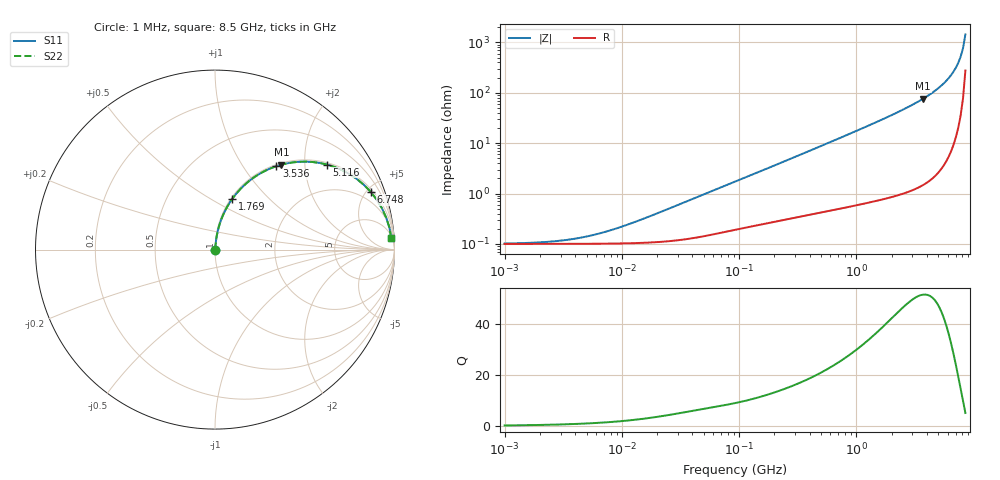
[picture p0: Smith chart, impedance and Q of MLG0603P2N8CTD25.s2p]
! S-Parameter Data Generated by TDK Corporation
! Copyright(C) 2025 TDK Corporation.
! All Rights Reserved.
! TDK P/N: MLG0603P2N8CTD25 (SMD / SMT Inductor (Coil))
! Property: L=2.8nH at 500MHz
! Size(LxWxT): 0.6x0.3x0.3mm
! Model Type: s2p (Touchstone File Format Version 1.0)
! Frequency: DC=Yes Start=1MHz Stop=8500MHz 198points Log-sweep
! Model Generated on Feb. 6, 2025
! Terms and conditions regarding TDK Simulation Models:
! 1)This simulation model is being provided solely for informational
!  purposes. Please refer to the specifications of the products in
!  terms of detailed characteristics of such products.
! 2)In no event shall TDK Corporation of any of its subsidiaries be
!  liable for any loss or damage arising, directly or indirectly,
!  from any information contained in this simulation model, including,
!  but not limited to loss or damages arising from any inaccuracies,
!  omissions or errors in connection with such information.
! 3)Any and all copyrights on this simulation model are owned by
!  TDK Corporation.  Duplication or redistribution of this simulation
!  model without prior written permission from TDK Corporation
!  is prohibited.
! 4)This simulation model is subject to any modification or change
!  without any prior notice.
! 5)Neither TDK Corporation nor any of its subsidiaries shall make any
!  warranty, express or implied, including but not limited to the
!  correctness, implied warranties of merchantability and fitness for
!  a particular purpose with respect to this simulation models.
! 6)The use of this simulation model shall be deemed to have consented
!  to the terms and conditions hereof.
! Port Assignments:
!  1 ---@@@--- 2
! Applicable Conditions:
!  Temperature = 25 degC
!  DC Bias Current = 0 A
!  Small Signal Operation
# Hz S MA R 50
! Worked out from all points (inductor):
!   197 points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, 1 MHz to 8.5 GHz, reference 50 ohm
!   read as one part in series: L = 3.1 nH near 16.71 MHz
!   highest Q = 51.7 at 3.703 GHz (marker M1), where L = 3.28 nH
!   S11 on the Smith chart (normalised r, x): 1 MHz: 1.00, +0.00; 1.769 GHz: 1.02, +0.63; 3.536 GHz: 1.03, +1.43; 5.116 GHz: 1.06, +2.59; 6.748 GHz: 1.19, +5.31; 8.5 GHz: 7, +28
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1000000  0.001018 11.1  0.999 -0.0  0.999 -0.0  0.001018 11.1
2403882  0.001105 25.1  0.999 -0.0  0.999 -0.0  0.001105 25.1
4587603  0.001346 41.7  0.999 -0.1  0.999 -0.1  0.001346 41.7
6337562  0.001597 50.8  0.999 -0.1  0.999 -0.1  0.001597 50.8
8755050  0.00199 59.2  0.999 -0.1  0.999 -0.1  0.00199 59.2
2.10461e7  0.004237 74.8  0.9989 -0.2  0.9989 -0.2  0.004237 74.8
9.219544e7  0.01721 82.7  0.998 -1.0  0.998 -1.0  0.01721 82.7
4.229561e8  0.07425 82.8  0.9934 -4.3  0.9934 -4.3  0.07425 82.8
9.270694e8  0.1595 78.8  0.9817 -9.2  0.9817 -9.2  0.1595 78.8
1.769233e9  0.2995 71.1  0.9466 -17.4  0.9466 -17.4  0.2995 71.1
1.940355e9  0.3275 69.5  0.937 -19.1  0.937 -19.1  0.3275 69.5
2.680511e9  0.4463 62.3  0.8856 -26.5  0.8856 -26.5  0.4463 62.3
3.535948e9  0.5766 53.7  0.8059 -35.2  0.8059 -35.2  0.5766 53.7
3.703002e9  0.6008 52.0  0.7878 -36.9  0.7878 -36.9  0.6008 52.0
4.453958e9  0.7035 44.2  0.6969 -44.7  0.6969 -44.7  0.7035 44.2
5.115526e9  0.7832 37.2  0.6052 -51.5  0.6052 -51.5  0.7832 37.2
5.87536e9  0.8597 29.3  0.4892 -59.3  0.4892 -59.3  0.8597 29.3
6.748056e9  0.9252 20.4  0.348 -67.6  0.348 -67.6  0.9252 20.4
7.400733e9  0.9581 13.9  0.2411 -73.1  0.2411 -73.1  0.9581 13.9
7.750377e9  0.9702 10.6  0.1847 -75.4  0.1847 -75.4  0.9702 10.6
8.116539e9  0.9791 7.3  0.1269 -76.9  0.1269 -76.9  0.9791 7.3
8.5e9  0.9846 3.8  0.06836 -75.1  0.06836 -75.1  0.9846 3.8
